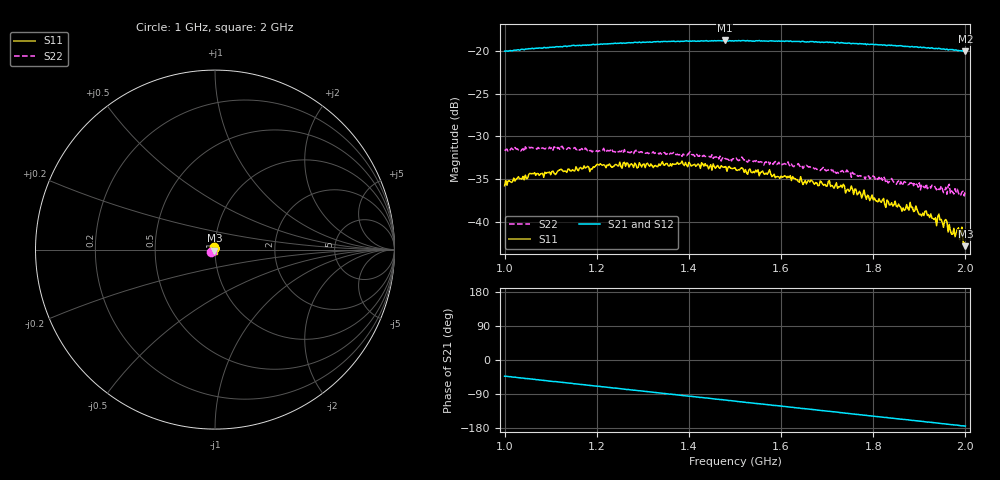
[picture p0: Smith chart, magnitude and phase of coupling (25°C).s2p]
!Agilent Technologies,E8363C,MY43030407,A.09.42.15
!Agilent E8363C: A.09.42.15
!Date: Friday, September 05, 2025 17:21:23
!Correction: S11(Full 2 Port(1,2))
!S21(Full 2 Port(1,2))
!S12(Full 2 Port(1,2))
!S22(Full 2 Port(1,2))
!S2P File: Measurements: S11, S21, S12, S22:
# Hz S  dB  R 50
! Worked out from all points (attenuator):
!   401 points, 1 GHz to 2 GHz, reference 50 ohm
!   highest |S21| = -18.76 dB at 1.478 GHz (marker M1); lowest = -20.1 dB at 2 GHz (marker M2)
!   lowest |S11| = -42.9 dB at 2 GHz (marker M3), VSWR 1.01, Z = 49.6 - j0.611 ohm
!   |S11| at or under -10 dB: start of sweep to end of sweep
!   |S22| runs from -37.0 to -31.1 dB; largest |S21 - S12| = 0.0017
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1e9  -35.78 106.1  -20.02 -42.8  -19.99 -42.6  -31.68 -144.9
1.06e9  -34.35 95.0  -19.67 -50.2  -19.72 -50.4  -31.32 -146.5
1.1675e9  -33.80 76.6  -19.34 -64.6  -19.32 -64.5  -31.42 -149.5
1.2625e9  -33.50 55.5  -19.08 -77.4  -19.04 -77.1  -31.88 -152.1
1.335e9  -33.23 41.9  -18.91 -86.8  -18.89 -86.3  -32.06 -154.6
1.38e9  -33.20 32.1  -18.89 -92.8  -18.91 -92.8  -32.14 -155.9
1.4775e9  -33.59 11.3  -18.76 -105.5  -18.77 -105.5  -32.55 -157.4
1.5e9  -33.67 9.3  -18.79 -108.5  -18.79 -108.3  -32.67 -157.2
1.6675e9  -35.22 -34.5  -18.90 -130.6  -18.90 -130.5  -33.62 -159.7
1.7325e9  -36.00 -49.8  -19.03 -139.1  -19.09 -139.2  -34.00 -160.2
1.745e9  -36.19 -53.1  -19.08 -140.8  -19.05 -140.8  -34.14 -157.9
1.7575e9  -36.81 -54.8  -19.11 -142.5  -19.14 -142.5  -34.41 -160.9
1.79e9  -37.00 -61.3  -19.21 -147.1  -19.18 -146.7  -34.64 -157.6
1.835e9  -38.03 -74.6  -19.31 -152.7  -19.33 -152.6  -35.29 -156.5
1.865e9  -38.38 -82.7  -19.45 -156.7  -19.41 -156.6  -35.52 -155.8
1.885e9  -38.28 -92.7  -19.47 -159.4  -19.51 -159.2  -35.30 -154.5
1.9325e9  -39.75 -98.2  -19.72 -165.8  -19.70 -165.6  -35.75 -151.4
1.945e9  -39.81 -102.2  -19.72 -167.2  -19.75 -167.1  -36.20 -151.8
1.96e9  -40.00 -106.7  -19.76 -169.4  -19.83 -169.3  -36.77 -148.0
1.9725e9  -41.43 -110.5  -19.82 -170.8  -19.89 -170.9  -36.53 -149.5
1.9875e9  -42.09 -114.5  -19.96 -172.8  -19.98 -172.9  -36.98 -146.4
2e9  -42.86 -121.2  -20.05 -174.4  -20.01 -174.2  -36.30 -145.8
